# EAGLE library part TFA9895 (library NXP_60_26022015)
Boosted class-D audio amplifier with speaker boost protection The TFA9895 is a high efficiency class-D audio amplifier with a sophisticated speaker boost protection algorithm that features multi-band compression. It can deliver 2.65 W (RMS; THD = 1 %) output power into a 4  speaker at a battery voltage of 3.6 V. The internal boost converter raises the supply voltage to 5.3 V, providing ample headroom for major improvements in sound quality. A safe working environment is provided for the speaker under all operating conditions. The TFA9895 maximizes acoustic output while ensuring diaphragm displacement and voice coil temperature do not exceed their rated limits. This function is based on a speaker box model that operates in all loudspeaker environments (e.g. free air, closed box or vented box). Furthermore, advanced signal processing ensures that the quality of the audio signal is never degraded by unwanted clipping or distortion in the amplifier or speaker. Unlike competing solutions, the adaptive sound maximizer algorithm uses feedback to accurately calculate both the temperature and the excursion, allowing the TFA9895 to adapt to changes in the acoustic environment. Internal intelligent DC-to-DC conversion boosts the supply rail to provide additional headroom and power output. The supply voltage is only raised when necessary. This precaution maximizes the output power of the class-D audio amplifier while limiting quiescent power consumption. The multi-band processing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
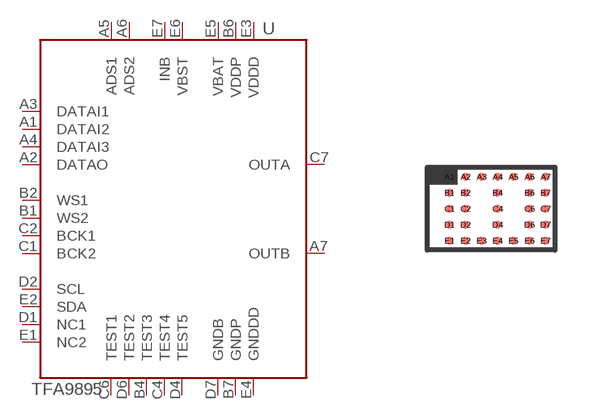
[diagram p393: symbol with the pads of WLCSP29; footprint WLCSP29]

Designator prefix U

## TFA9895  [WLCSP29]
A1  DATAI2  in
A2  DATAO  out
A3  DATAI1  in
A4  DATAI3  in
A5  ADS1  in
A6  ADS2  in
A7  OUTB  out
B1  WS2  in
B2  WS1  in
B4  TEST3  in
B6  VDDP  pwr
B7  GNDP  pwr
C1  BCK2  in
C2  BCK1  in
C4  TEST4  in
C6  TEST1  in
C7  OUTA  out
D1  NC1
D2  SCL
D4  TEST5  in
D6  TEST2  in
D7  GNDB  pwr
E1  NC2
E2  SDA
E3  VDDD  pwr
E4  GNDDD  pwr
E5  VBAT  pwr
E6  VBST  pwr
E7  INB  pwr

## Footprint WLCSP29 (pad centres in mm)
based on Intersil Technical Brief 451
smd 0.2 x 0.2: A1 -1.04,0.797; A2 -0.639,0.797; A3 -0.239,0.797; A4 0.161,0.797; A5 0.56,0.797; A6 0.961,0.797; A7 1.361,0.797; B1 -1.04,0.398; B2 -0.639,0.398; B4 0.161,0.398; B6 0.961,0.398; B7 1.361,0.398; C1 -1.04,-0.003; C2 -0.639,-0.003; C4 0.161,-0.003; C6 0.961,-0.003; C7 1.361,-0.003; D1 -1.04,-0.403; D2 -0.639,-0.403; D4 0.161,-0.403; D6 0.961,-0.403; D7 1.361,-0.403; E1 -1.04,-0.802; E2 -0.639,-0.802; E3 -0.239,-0.802; E4 0.161,-0.802; E5 0.56,-0.802; E6 0.961,-0.802; E7 1.361,-0.802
